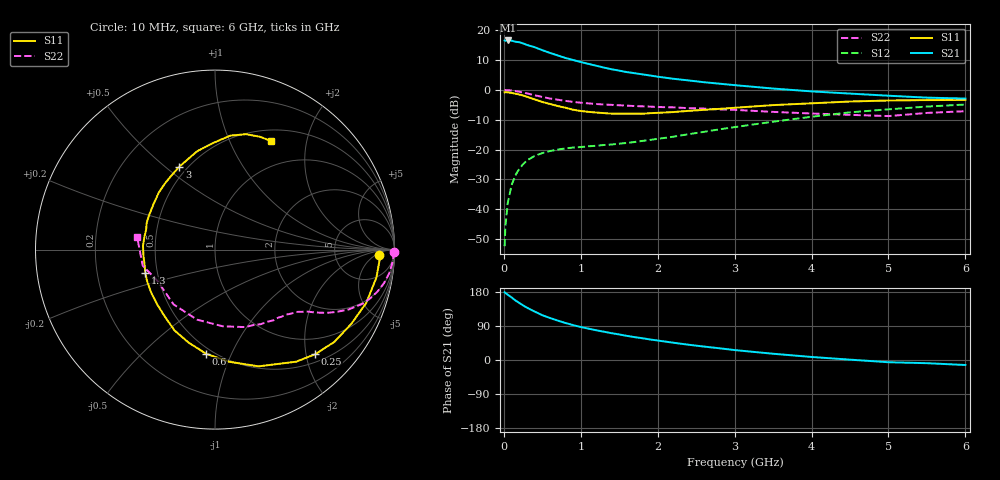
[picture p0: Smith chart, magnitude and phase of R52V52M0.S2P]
! SIEMENS Small Signal Semiconductors
! BFR183
! Si NPN RF Bipolar Junction Transistor in SOT23
! VCE = 2.5 V  IC = 2 mA
! Common Emitter S-Parameters:  May  1996
# GHz  S  MA  R  50
!  f  S11  S21  S12  S22
! GHz  MAG  ANG  MAG  ANG  MAG  ANG  MAG  ANG
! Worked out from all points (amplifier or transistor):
!   36 points, 10 MHz to 6 GHz, reference 50 ohm
!   highest |S21| = 16.6 dB at 50 MHz (marker M1)
!   |S21| within 3 dB of that: start of sweep to 473.9 MHz
!   unconditionally stable (mu >= 1): 1.371 GHz to 2.853 GHz
!   at 250 MHz: K = 0.23, MSG = 20.3 dB, |S12| = -24.9 dB
!   at 1.4 GHz: K = 1.02, MAG = 11.8 dB, |S12| = -18.3 dB
!   at 6 GHz: K = 0.92, MSG = 1.0 dB, |S12| = -4.9 dB
!   S11 on the Smith chart (normalised r, x): 10 MHz: 19, -7; 250 MHz: 0.65, -2.18; 600 MHz: 0.46, -0.81; 1.3 GHz: 0.43, -0.14; 3 GHz: 0.45, +0.56; 6 GHz: 0.64, +1.44
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0.01  0.9135 -2.0  6.761 178.9  0.0024 93.4  0.9972 -0.7
0.02  0.9188 -3.7  6.666 176.9  0.0051 84.1  0.9956 -1.6
0.05  0.9128 -9.8  6.771 172.5  0.0126 85.3  0.992 -4.0
0.1  0.8938 -19.3  6.727 165.3  0.0252 79.2  0.9792 -7.8
0.15  0.865 -28.5  6.447 157.3  0.037 73.7  0.9594 -11.3
0.2  0.8406 -37.7  6.334 150.6  0.0475 69.3  0.9341 -14.6
0.25  0.807 -46.3  6.045 144.1  0.0568 64.8  0.9039 -17.7
0.3  0.7709 -54.1  5.704 138.1  0.0658 61.2  0.8766 -20.1
0.4  0.6944 -69.5  5.221 127.9  0.0782 55.2  0.8177 -24.0
0.5  0.6295 -82.9  4.651 118.2  0.0874 50.3  0.7621 -27.1
0.6  0.5823 -94.9  4.183 110.8  0.0946 47.0  0.7191 -29.3
0.8  0.5037 -116.6  3.446 97.8  0.1047 42.8  0.6568 -32.2
0.9  0.4669 -126.6  3.183 92.1  0.1082 42.3  0.6319 -33.3
1.1  0.4299 -145.3  2.74 82.8  0.1136 42.2  0.5957 -35.6
1.3  0.4096 -161.3  2.376 74.7  0.1194 43.3  0.5706 -37.5
1.7  0.3997 170.0  1.912 60.4  0.1341 47.5  0.5374 -42.4
2.2  0.426 143.7  1.544 45.7  0.1643 52.2  0.5113 -50.4
3  0.503 113.3  1.205 26.2  0.2384 53.3  0.4638 -68.6
3.5  0.5575 100.2  1.057 16.5  0.2935 49.8  0.4292 -84.3
4.5  0.6405 82.4  0.87 0.9  0.4219 37.8  0.3829 -127.1
5.5  0.6767 68.2  0.744 -8.4  0.5268 23.2  0.4125 -167.4
6  0.681 62.6  0.718 -13.2  0.5703 14.0  0.4404 170.5
